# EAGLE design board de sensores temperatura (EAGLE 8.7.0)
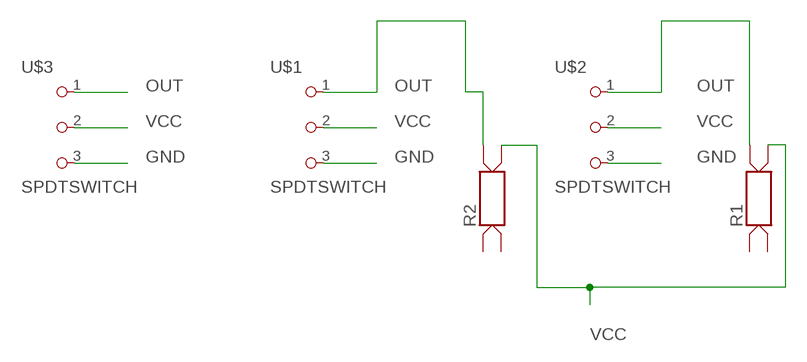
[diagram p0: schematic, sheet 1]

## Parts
R1  R-MELF0207  [MELF0207]
R2  R-MELF0207  [MELF0207]
U$1  SPDTSWITCH  [SPDTSWITCH]
U$2  SPDTSWITCH  [SPDTSWITCH]
U$3  SPDTSWITCH  [SPDTSWITCH]

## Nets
GND: U$1.3 U$2.3 U$3.3
OUT: R1.1B(PT100-B1) R2.1B(PT100-B1) U$1.1 U$2.1 U$3.1
VCC: R1.2B(PT100-B2) R2.2B(PT100-B2) U$1.2 U$2.2 U$3.2
Unconnected: R1.1A(PT100-A1) R1.2A(PT100-A2) R2.1A(PT100-A1) R2.2A(PT100-A2)

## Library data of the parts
R1 R2 = resistor-ruf:R-MELF0207: 4-pole RESISTOR; MPN: CMB 0207 2% B2 470K; OC_FARNELL: 1505905; OC_NEWARK: 15R0802
U$1-U$3 = fab:SPDTSWITCH

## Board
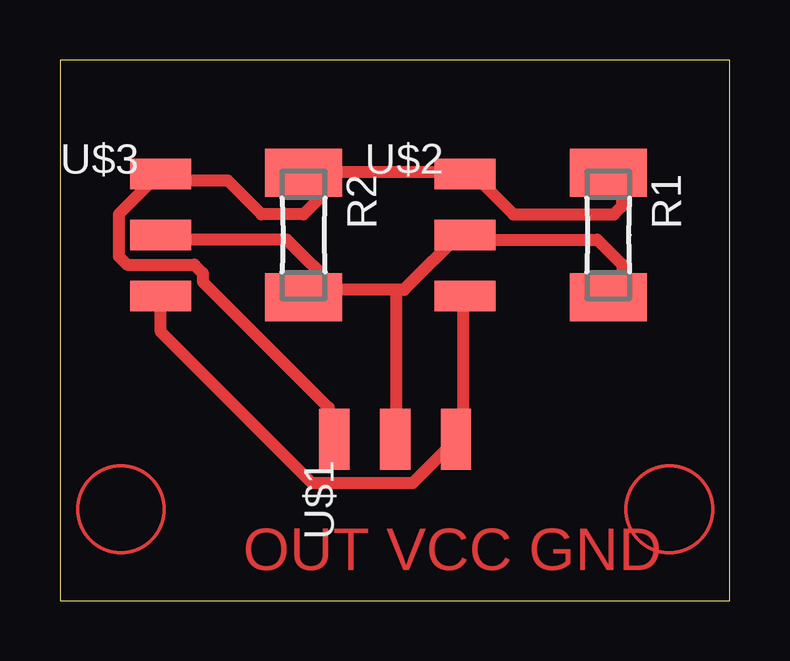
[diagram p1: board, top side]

Size 27.92 x 22.53 mm. Coordinates in mm from the lower left corner, seen from the top.
Outline: 0,0 27.92,0 27.92,22.53 0,22.53 0,0
Copper layers (1*16): Top 0.035mm / dielectric 1.5mm / Bottom 0.035mm
Design rules "default *": minimum track width 0.5mm, minimum drill 0.5mm, track to track 0.2mm, track to pad 0.2mm, pad to pad 0.2mm, via to via 0.2mm, smd to smd 0.2mm, copper to edge 40mil, drill to drill 6mil, minimum pad ring 10mil, minimum via ring 8mil, stop-mask expansion 4mil, vias tented up to drill 0mil, thermal gap 10mil

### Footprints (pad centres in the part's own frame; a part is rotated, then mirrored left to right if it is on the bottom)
MELF0207 = smd 2 x 1.6: 1A -2.6,-0.8; 1B -2.6,0.8; 2A 2.6,-0.8; 2B 2.6,0.8
SPDTSWITCH = smd 2.54 x 1.27: 1 0.38,2.54; 2 0.38,0; 3 0.38,-2.54

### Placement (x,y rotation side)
R1  22.86,15.24 270 top
R2  10.16,15.24 270 top
U$1  13.97,6.35 90 top
U$2  16.51,15.24 0 top
U$3  3.81,15.24 0 top

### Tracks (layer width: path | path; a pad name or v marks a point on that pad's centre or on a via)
GND
  Top 0.5: U$2.3 16.8,12.6 16.8,7 U$1.3 16.45,6.65 14.7,4.9 10.5,4.9 4.2,11.2 4.2,12.6 U$3.3
OUT
  Top 0.5: R1.1B 23.45,17.5 23.45,16.45 23.1,16.1 18.9,16.1 17.15,17.85 U$2.1 16.8,17.85 11.2,17.85 R2.1B 10.85,17.5 10.85,16.8 10.15,16.1 8.4,16.1 7,17.5 4.2,17.5 U$3.1 3.85,17.5 2.45,16.1 2.45,14.35 2.8,14 5.6,14 5.95,13.65 5.95,13.3 11.2,8.05 11.2,7 U$1.1
VCC
  Top 0.5: 14,12.95 14.35,12.95 16.8,15.4 U$2.2 17.15,15.05 22.4,15.05 23.45,14 23.45,12.95 R1.2B | 14,12.95 11.55,12.95 | 11.55,12.95 11.2,12.95 R2.2B 11.55,12.95 | 14,12.95 14,7 U$1.2 | 11.55,12.95 9.45,15.05 4.2,15.05 U$3.2
(copper drawn outside any net)
  shapes: Top circle x2

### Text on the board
Top: OUT VCC GND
